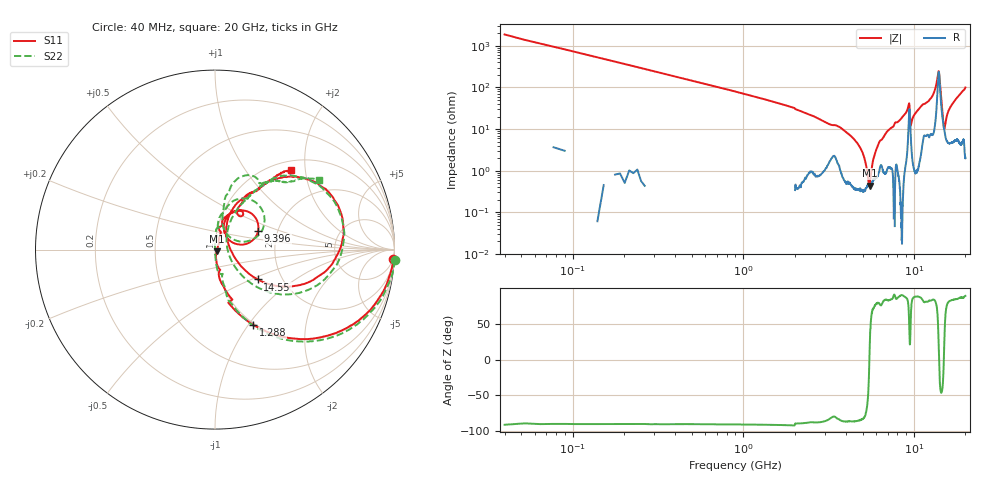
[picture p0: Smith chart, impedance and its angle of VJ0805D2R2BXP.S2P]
! VJ0805D2R2BXP
! DATE 10/29/2021  11:35
! CAPACITORS MOUNTED IN SERIES ON 25 MIL THICK MICROSTRIP SUBSTRATE
# GHz  S  MA  R  50.00
!  FREQ  S11M  S11A  S21M  S21A  S12M  S12A  S22M  S22A
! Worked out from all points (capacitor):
!   1601 points, 40 MHz to 20 GHz, reference 50 ohm
!   read as one part in series: C = 2.16 pF near 139.8 MHz
!   lowest |Z| = 440 mohm at 5.492 GHz (marker M1)
!   series resonance near 5.477 GHz, so ESL is about 390 pH
!   S11 on the Smith chart (normalised r, x): 40 MHz: 4, -36; 1.288 GHz: 0.98, -1.05; 9.396 GHz: 1.58, +0.36; 14.55 GHz: 1.51, -0.55; 20 GHz: 1.18, +1.69
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0.04  0.9946 -3.2  0.05356 87.7  0.05683 86.9  1.003 -3.4
0.21465  0.9546 -16.1  0.2801 73.5  0.2802 73.7  0.9666 -16.5
0.41425  0.8651 -29.4  0.4925 60.5  0.4922 60.5  0.8777 -29.9
1.2875  0.4698 -63.0  0.8841 28.3  0.8836 28.3  0.4896 -62.2
3.370825  0.1177 -76.0  0.9693 6.2  0.969 6.2  0.1424 -73.0
5.00505  0.03474 -81.1  0.9964 1.0  0.9951 1.0  0.03807 -86.2
5.491575  0.01348 -50.7  0.9952 -0.6  0.9954 -0.7  0.009248 -94.2
5.65375  0.01086 -8.4  0.9955 -1.2  0.9947 -1.2  0.001373 166.3
5.840875  0.01524 27.9  0.9942 -1.8  0.9933 -1.8  0.01237 89.8
6.05295  0.02587 50.5  0.9931 -2.6  0.9936 -2.6  0.02482 90.4
6.70165  0.05924 68.5  0.9905 -4.6  0.9899 -4.6  0.05565 84.2
9.39625  0.262 23.5  0.7568 -11.5  0.7564 -11.6  0.3061 26.8
9.59585  0.09718 50.5  0.9439 -7.0  0.9431 -7.1  0.1113 56.5
10.02  0.187 69.7  0.9706 -13.0  0.9699 -13.1  0.202 77.9
12.14075  0.3314 60.5  0.8673 -24.6  0.8663 -24.7  0.4457 52.8
13.35083  0.6384 38.5  0.6737 -41.6  0.673 -41.7  0.6281 40.0
13.9621  0.7087 3.1  0.2898 -12.9  0.2895 -13.0  0.7078 -0.4
14.54842  0.2908 -34.9  0.7629 10.2  0.7626 10.1  0.3132 -41.7
15.07237  0.08102 12.2  0.9106 -4.2  0.9102 -4.3  0.0688 10.5
15.67117  0.1681 66.3  0.9324 -13.7  0.9318 -13.8  0.2063 61.7
16.68165  0.295 63.8  0.9013 -22.5  0.9012 -22.6  0.3417 57.8
20  0.6155 46.3  0.6978 -50.2  0.6965 -50.5  0.6971 33.9
